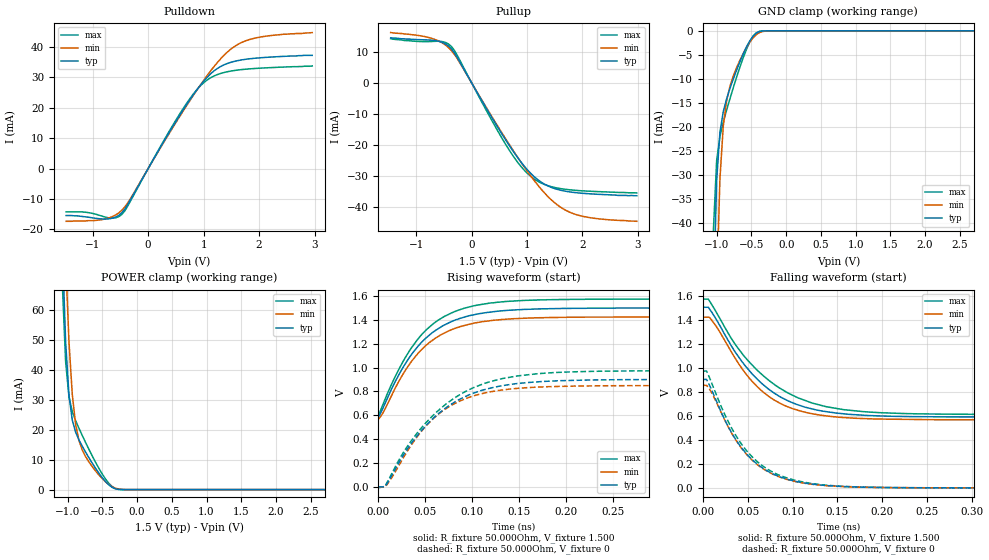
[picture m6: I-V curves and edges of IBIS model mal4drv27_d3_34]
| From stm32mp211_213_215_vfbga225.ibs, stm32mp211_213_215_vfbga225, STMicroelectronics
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[Model] mal4drv27_d3_34
Model_type   I/O
Polarity   Non-Inverting
Enable   Active-High
C_comp   1.653pF   1.649pF   1.658pF
C_comp_pullup   821.240fF   815.174fF   828.427fF
C_comp_pulldown 737.945fF   733.914fF   744.436fF
Vinh = 885.000mV
Vinl = 615.000mV
Vmeas = 750.000mV
Vref = 750.000mV
Rref = 50Ohms
Cref = 0pF
[Model Spec]
Vinh   885.000mV   848.000mV   923.000mV
Vinl   615.000mV   578.000mV   653.000mV
Vmeas   750.000mV   713.000mV   788.000mV
Vref   750.000mV   713.000mV   788.000mV
D_overshoot_ampl_h 0.4 NA   NA
D_overshoot_ampl_l 0.4 NA   NA
D_overshoot_area_l 100.000m NA   NA
D_overshoot_area_h 100.000m NA   NA
[Receiver Thresholds]
Vth = 750.000mV
Vth_min = 713.000mV
Vth_max = 788.000mV
Vinh_ac = 135.000mV
Vinh_dc = 100.000mV
Vinl_ac = -135.000mV
Vinl_dc = -100.000mV
Tslew_ac = 5.000ns
Threshold_sensitivity = 0.5
Reference_supply Pullup_ref
[Temperature Range]   25.000   125.000   -40.000
[Voltage Range]   1.500V   1.425V   1.575V
[GND Clamp Reference]   0.00V   0.00V   0.00V
[C Comp Corner]
| variable   typ   min   max
C_comp 1.658pF   1.653pF   1.649pF
C_comp_pullup 821.240fF   828.427fF   815.174fF
C_comp_pulldown 733.914fF   744.436fF   737.945fF
[Pulldown Reference]   0.00V   0.00V   0.00V
[POWER Clamp Reference]   1.500V   1.425V   1.575V
[Pullup Reference]   1.500V   1.425V   1.575V
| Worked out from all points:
|   slope of the pulldown table from 0 to 0.225 V, typ, clamps not added: 31.6 ohm
|   slope of the pullup table from 0 to 0.225 V, typ, clamps not added: 32.2 ohm
|   GND clamp passes 1 mA (typ) near -0.47 V on its own axis
|   POWER clamp passes 1 mA (typ) near -0.37 V on its own axis
|   rising waveform, R_fixture 50.000Ohm, V_fixture 1.500: 20-80 % time 50.7ps typ, 49.5ps min, 50ps max; typ from 0.586 V to 1.5 V
|   rising waveform, R_fixture 50.000Ohm, V_fixture 0: 20-80 % time 63ps typ, 55.7ps min, 68.4ps max; typ from 0 V to 0.901 V
|   falling waveform, R_fixture 50.000Ohm, V_fixture 1.500: 20-80 % time 61.8ps typ, 55.6ps min, 70.5ps max; typ from 1.51 V to 0.592 V
|   falling waveform, R_fixture 50.000Ohm, V_fixture 0: 20-80 % time 48.7ps typ, 47.8ps min, 49.9ps max; typ from 0.906 V to 0 V
[GND Clamp]
-1.48V    -1.356A    -1.372A    -1.368A
-1.05V    -57.52mA   -98.82mA   -41.99mA
-1.002V   -31.12mA   -53.93mA   -27.05mA
-954.6mV  -21.13mA   -30.8mA    -21.99mA
-906.8mV  -16.83mA   -19.93mA   -19.06mA
-859.1mV  -14.2mA    -14.62mA   -16.56mA
-763.6mV  -10.09mA   -9.457mA   -11.91mA
-668.2mV  -6.482mA   -6.16mA    -7.611mA
-525mV    -2.097mA   -2.366mA   -2.333mA
-429.5mV  -449.8uA   -771.1uA   -394uA
-238.6mV  -1.709uA   -14.74uA   -370nA
2.959V    53.06nA    707.1nA    76.78nA
[Power Clamp]
-1.459V   570.2mA    591.8mA    567.2mA
-1.077V   80.71mA    114.2mA    68.27mA
-1.03V    49.21mA    76.71mA    42.66mA
-981.8mV  31.4mA     49.26mA    30.9mA
-934.1mV  23.16mA    31.72mA    25.95mA
-886.4mV  19.16mA    21.79mA    22.98mA
-838.6mV  16.6mA     16.39mA    20.46mA
-743.2mV  12.52mA    11.03mA    15.74mA
-647.7mV  8.857mA    7.696mA    11.27mA
-361.4mV  773.2uA    986uA      1.034mA
-218.2mV  12.39uA    63.5uA     9.952uA
2.98V     -55.08nA   -1.144uA   -55.82nA
[Pulldown]
-1.48V    -15.5mA    -17.4mA    -14.3mA
-1.098V   -16mA      -17.2mA    -14.48mA
-763.6mV  -16.66mA   -16.57mA   -16.07mA
-477.3mV  -14.6mA    -13.79mA   -15.17mA
-334.1mV  -10.79mA   -10.35mA   -11.23mA
286.4mV   9.026mA    8.776mA    9.336mA
715.9mV   21.66mA    21.36mA    22.07mA
1.002V    28.8mA     29.08mA    28.29mA
1.241V    32.88mA    34.77mA    30.9mA
1.527V    35.18mA    39.84mA    32.22mA
1.814V    36.13mA    42.42mA    32.81mA
2.959V    37.3mA     44.8mA     33.8mA
[Pullup]
-1.459V   14.5mA     16.2mA     14.21mA
-743.2mV  13.77mA    14.46mA    13.3mA
-504.6mV  12.86mA    12.59mA    13.2mA
-361.4mV  10.89mA    10.33mA    11.64mA
402.3mV   -12.32mA   -12.01mA   -13.35mA
688.6mV   -20.49mA   -20.17mA   -22.01mA
927.3mV   -26.43mA   -26.59mA   -27.79mA
1.166V    -30.9mA    -32.42mA   -31.53mA
1.5V      -34.2mA    -38.79mA   -33.84mA
1.834V    -35.42mA   -42.27mA   -34.69mA
2.264V    -36.02mA   -43.9mA    -35.15mA
2.98V     -36.5mA    -44.76mA   -35.6mA
[Ramp]
R_load=50.000Ohm
dV/dt_r   542.760mV/57.500ps  511.948mV/53.000ps  580.890mV/60.500ps
dV/dt_f   542.760mV/56.000ps  511.949mV/52.500ps  580.890mV/61.000ps
[Rising waveform]
R_fixture=50.000Ohm
V_fixture=1.500
V_fixture_min=1.425
V_fixture_max=1.575
0s        585.7mV    566.5mV    601.3mV
6ps       680.1mV    636.2mV    712.8mV
22ps      943.3mV    888.4mV    989mV
32ps      1.074V     1.017V     1.128V
43ps      1.187V     1.126V     1.249V
63ps      1.325V     1.259V     1.395V
91ps      1.423V     1.353V     1.498V
127ps     1.474V     1.401V     1.549V
172ps     1.493V     1.419V     1.569V
469ps     1.5V       1.425V     1.575V
[Rising waveform]
R_fixture=50.000Ohm
V_fixture=0
0s        -283.2uV   -1.851mV   -8.702mV
9ps       23.93mV    16.82mV    31.7mV
33ps      342.4mV    326.5mV    364.4mV
46ps      473.6mV    467.5mV    496.6mV
62ps      601.2mV    596.9mV    627.6mV
86ps      732.7mV    717.7mV    770mV
119ps     828.3mV    797mV      883mV
165ps     878.9mV    835.3mV    946.5mV
207ps     893.6mV    845.2mV    965.3mV
476ps     900.9mV    849.7mV    974.4mV
[Falling waveform]
R_fixture=50.000Ohm
V_fixture=1.500
V_fixture_min=1.425
V_fixture_max=1.575
0s        1.508V     1.425V     1.576V
6ps       1.508V     1.425V     1.576V
9ps       1.477V     1.409V     1.541V
38ps      1.113V     1.058V     1.178V
66ps      869.1mV    807.1mV    944.6mV
91ps      741mV      688.1mV    809mV
121ps     660.5mV    620mV      709.8mV
156ps     619.1mV    587.5mV    654mV
216ps     597.2mV    571.7mV    622.1mV
475ps     591.7mV    568.2mV    613.1mV
[Falling waveform]
R_fixture=50.000Ohm
V_fixture=0
0s        905.5mV    856.2mV    975.8mV
4ps       905.5mV    856.2mV    975.8mV
8ps       847.7mV    817.1mV    908.2mV
29ps      501.1mV    497.9mV    542.1mV
50ps      272.6mV    268.5mV    298.7mV
73ps      136.1mV    133.1mV    151.7mV
104ps     52.92mV    50.76mV    60.27mV
135ps     20.58mV    19.35mV    23.66mV
192ps     3.554mV    3.346mV    4.189mV
473ps     0V         5.368uV    0V
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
